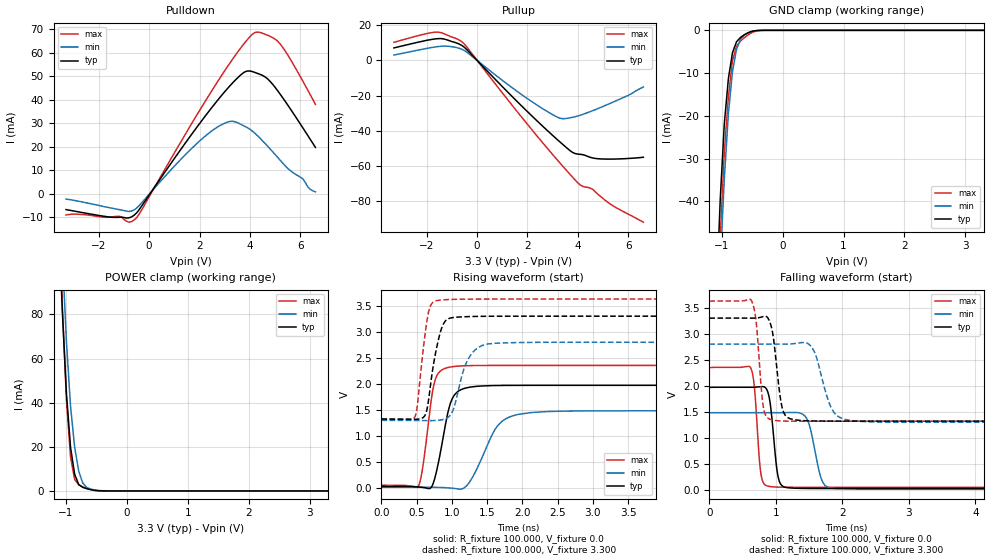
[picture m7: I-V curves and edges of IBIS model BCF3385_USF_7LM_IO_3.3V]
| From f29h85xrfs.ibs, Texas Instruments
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|BCF3385_USF_7LM_IO_3.3V;
|   Model BCF3385_USF_7LM_IO_3.3V
[Model]   BCF3385_USF_7LM_IO_3.3V
Model_type   I/O
Polarity   Non-Inverting
Enable   Active-Low
Vinl =   0.800V
Vinh =   2.000V
Vmeas =  1.650V
Cref =   15.000pF
Vref =   0.0V
|   typ   min   max
C_comp   0.611pF   0.603pF   0.631pF
[Model Spec]
Vinh   2.000V   2.000V   2.000V
Vinl   0.800V   0.800V   0.800V
[Temperature Range]   25   155   -40
[Voltage Range]   3.300V   2.800V   3.630V
[Pullup Reference]   3.300V   2.800V   3.630V
[Pulldown Reference]   0.0V   0.0V   0.0V
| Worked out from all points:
|   slope of the pulldown table from 0 to 0.495 V, typ, clamps not added: 63.8 ohm
|   slope of the pullup table from 0 to 0.495 V, typ, clamps not added: 66.6 ohm
|   GND clamp passes 1 mA (typ) near -0.62 V on its own axis
|   POWER clamp passes 1 mA (typ) near -0.65 V on its own axis
|   rising waveform, R_fixture 100.000, V_fixture 0.0: 20-80 % time 171ps typ, 314ps min, 132ps max; typ from 0.019 V to 1.97 V
|   rising waveform, R_fixture 100.000, V_fixture 3.300: 20-80 % time 147ps typ, 201ps min, 115ps max; typ from 1.32 V to 3.3 V
|   falling waveform, R_fixture 100.000, V_fixture 0.0: 20-80 % time 90ps typ, 145ps min, 74.4ps max; typ from 1.97 V to 0.019 V
|   falling waveform, R_fixture 100.000, V_fixture 3.300: 20-80 % time 109ps typ, 204ps min, 84.3ps max; typ from 3.3 V to 1.32 V
[Pulldown]
|Voltage   I(typ)   I(min)   I(max)
-3.3V     -6.702mA   -2.223mA   -8.98mA
-1.2V     -9.981mA   -6.684mA   -9.543mA
-900mV    -10.31mA   -7.355mA   -11.63mA
-500mV    -8.146mA   -6.096mA   -10.17mA
1.5V      22.57mA    17.34mA    26.52mA
2.7V      39.6mA     28.35mA    47.49mA
3.3V      47.08mA    30.9mA     57.15mA
3.8V      51.94mA    28.7mA     64.36mA
4.2V      51.67mA    25.76mA    68.68mA
4.7V      48.95mA    20.31mA    67.5mA
5.2V      42.43mA    14.31mA    63.81mA
6.6V      19.75mA    845.5uA    38.08mA
[Pullup]
|Voltage   I(typ)   I(min)   I(max)
-3.3V     7.098mA    3.077mA    10.29mA
-1.6V     12.34mA    7.784mA    16.12mA
-1.3V     12.15mA    8.165mA    15.13mA
-600mV    8.475mA    6.298mA    10.58mA
1.9V      -27.79mA   -20.8mA    -34.64mA
2.7V      -38.76mA   -28.36mA   -48.54mA
3.3V      -46.57mA   -32.96mA   -58.58mA
3.8V      -52.49mA   -32.38mA   -66.65mA
4.1V      -53.5mA    -31.2mA    -70.99mA
4.6V      -55.6mA    -28.58mA   -73.51mA
5.3V      -56.21mA   -24.36mA   -81.93mA
6.6V      -55.16mA   -15.13mA   -92.14mA
[GND_clamp]
|Voltage   I(typ)   I(min)   I(max)
-3.3V     -1.213A    -1.056A    -1.445A
-1.089V   -64.21mA   -77.86mA   -77.8mA
-1.022V   -39.64mA   -54.82mA   -48.63mA
-955mV    -21.9mA    -34.83mA   -28.71mA
-888mV    -11.29mA   -19.46mA   -15.61mA
-821mV    -5.25mA    -9.624mA   -7.075mA
-754mV    -2.66mA    -4.381mA   -3.721mA
-687mV    -1.623mA   -2.024mA   -2.474mA
-553mV    -494.7uA   -494.4uA   -941.5uA
-419mV    -39.5uA    -64.26uA   -130.3uA
-285mV    -654.2nA   -3.515uA   -2.378uA
3.3V      0A         0A         0A
[POWER_clamp]
|Voltage   I(typ)   I(min)   I(max)
-3.3V     1.958A     2.188A     2.116A
-1.122V   125.8mA    154.1mA    133.8mA
-1.055V   81.17mA    107.1mA    83.43mA
-988mV    44.06mA    67.53mA    41.21mA
-921mV    19.7mA     38.38mA    15.37mA
-854mV    7.614mA    19.9mA     5.213mA
-787mV    2.907mA    8.995mA    2.715mA
-720mV    1.618mA    3.529mA    1.849mA
-653mV    1.007mA    1.525mA    1.161mA
-586mV    551.9uA    788.6uA    599.1uA
-385mV    14.09uA    57.25uA    8.652uA
3.3V      0A         0A         0A
[Ramp]
| variable   typ   min   max
dV/dt_r   1.169/0.171n   0.883/0.313n   1.385/0.132n
dV/dt_f   1.189/0.109n   0.904/0.203n   1.388/84.551p
R_load = 100.000
[Rising Waveform]
R_fixture= 100.000
V_fixture= 0.0
V_fixture_min= 0.0
V_fixture_max= 0.0
|time   V(typ)   V(min)   V(max)
0s        19.42mV    7.367mV    43.89mV
529ps     11.25mV    8.017mV    40.7mV
589ps     2.389mV    7.972mV    416mV
703ps     -686.1uV   6.599mV    1.653V
758ps     185.9mV    5.152mV    2.053V
980ps     1.629V     -8.538mV   2.321V
1.224ns   1.925V     60.22mV    2.347V
1.706ns   1.966V     1.272V     2.351V
2.126ns   1.968V     1.445V     2.352V
10ns      1.969V     1.479V     2.352V
[Rising Waveform]
R_fixture= 100.000
V_fixture= 3.300
V_fixture_min= 2.800
V_fixture_max= 3.630
|time   V(typ)   V(min)   V(max)
0s        1.317V     1.293V     1.315V
476ps     1.315V     1.292V     1.366V
511ps     1.317V     1.292V     1.59V
614ps     1.382V     1.29V      2.899V
667ps     1.673V     1.289V     3.371V
805ps     2.826V     1.295V     3.604V
938ps     3.241V     1.346V     3.618V
1.226ns   3.291V     2.462V     3.627V
1.504ns   3.297V     2.763V     3.628V
10ns      3.299V     2.799V     3.628V
[Falling Waveform]
R_fixture= 100.000
V_fixture= 0.0
V_fixture_min= 0.0
V_fixture_max= 0.0
|time   V(typ)   V(min)   V(max)
0s        1.968V     1.479V     2.351V
623ps     1.968V     1.479V     2.339V
676ps     1.969V     1.479V     1.99V
771ps     1.979V     1.479V     342.2mV
901ps     1.767V     1.479V     60.33mV
1.032ns   255.8mV    1.479V     47.23mV
1.158ns   39.01mV    1.48V      44.7mV
1.458ns   21.45mV    1.379V     43.88mV
1.827ns   19.95mV    29.02mV    43.83mV
10ns      19.38mV    7.384mV    43.81mV
[Falling Waveform]
R_fixture= 100.000
V_fixture= 3.300
V_fixture_min= 2.800
V_fixture_max= 3.630
|time   V(typ)   V(min)   V(max)
0s        3.299V     2.799V     3.628V
636ps     3.299V     2.799V     3.628V
705ps     3.301V     2.799V     3.215V
816ps     3.332V     2.799V     1.557V
961ps     2.939V     2.799V     1.335V
1.101ns   1.543V     2.799V     1.319V
1.283ns   1.342V     2.808V     1.315V
1.883ns   1.318V     1.469V     1.315V
2.203ns   1.317V     1.317V     1.315V
10ns      1.317V     1.293V     1.315V
